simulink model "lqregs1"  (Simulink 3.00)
settings: Solver=ode45  StartTime=0.0  StopTime=10.0  RelTol=1e-3

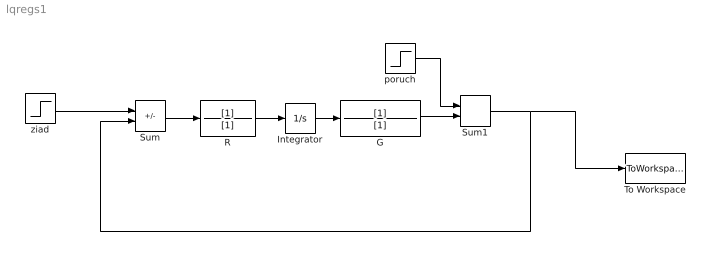
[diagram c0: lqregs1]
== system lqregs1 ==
  G : TransferFcn  Numerator=[1]  Denominator=[1]
  Integrator : Integrator  ExternalReset=none  InitialConditionSource=internal  InitialCondition=0  LimitOutput=off  UpperSaturationLimit=inf  LowerSaturationLimit=-inf  ShowSaturationPort=off  ShowStatePort=off  AbsoluteTolerance=auto
  R : TransferFcn  Numerator=[1]  Denominator=[1]
  Sum : Sum  Inputs=+-  SaturateOnIntegerOverflow=on
  Sum1 : Sum  Inputs=++  SaturateOnIntegerOverflow=on
  To Workspace : ToWorkspace  VariableName=y  SampleTime=-1  SaveFormat=Matrix
  poruch : Step  Time=50  Before=0  After=2  SampleTime=0
  ziad : Step  Time=0  Before=0  After=5  SampleTime=0
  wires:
  R/1 -> Integrator/1
  Integrator/1 -> G/1
  Sum/1 -> R/1
  ziad/1 -> Sum/1
  G/1 -> Sum1/2
  poruch/1 -> Sum1/1
  Sum1/1 -> Sum/2, To Workspace/1
